|   IBIS model for TI tms320c6657_55 DSP
[IBIS Ver]   5.0
[Disclaimer]   Please be aware that in the absence of a written agreement
|   Texas Instruments(TI) assumes no liability for:
|   (1) The accuracy of the IBIS models provided to your company,
|   however, the IBIS model is compliant to industry standard
|   IQ Level 2a.  Refer to IBIS Quality Section below for
|   for full details.
|   (2) The proper functioning of these Models in your design
|   or for any resulting applications
|   (3) Infringement of patents, copyrights or intellectual
|   property rights resulting from your use of these
|   models.
|   TI provides IBIS Models as a service to our customers and
|   therefore reserves the right to limit distribution of the
|   Models.  The information is subject to change without notice.
[File Name]  tms320c6657_55_r1p2.ibs
[File Rev]   1.2
[Date]   18Sept2012
[Source]   Texas Instruments Incorporated
[Copyright]   Property of Texas Instruments Incorporated.
|   Unauthorized reproduction and/or distribution is strictly.
|   prohibited.
|   This product is protected under copyright law and trade
|   secret law as an unpublished work.
|   Created 2012,(C) Copyright 2010-2020,
|   Texas Instruments Incorporated., All Rights Reserved.
|   These commodities are under the U.S. Government
|   distribution license control. As such,they are not to be
|   re-exported without the prior approval of the U.S.
|   Department of Commerce.
[Notes]
   For SerDes simulations use Texas Instruments IBIS AMI models
   Some IV curves contain Non monotonic data points.
|   Model Generated by W.T.
|   Model Updated by R.L.
|   **For SerDes simulations use Texas Instruments IBIS AMI models**
| The DDR3
| Definitions:
| Drive strength defined by resistor value connected to PTV15 pin
|   9MA_FT9MA   : Full Termination Thevenin  [45 ohm] [45ohm to Vtt]
| Slew Rate Definitions:
| The Driver Slew Rate is defined by the value of the DDRSLRATE0 and
| DDRSLRATE1 pins.
|   FASTEST Slew Rate : SR1 0;SR0 0
|   FAST Slew Rate   : SR1 0;SR0 1
|   SLOW Slew Rate   : SR1 1;SR0 0
|   SLOWEST Slew Rate : SR1 1;SR0 1
| To choose the correct model, determine the settings of the DDRSLRATE[1:0]
| pins.  Look for the keyword from the tables above to select the proper
| models.  For example if the DDRSLRATE1 pin is pulled high and the
| DDRSLRATE0 pin is pulled low then the slew rate keyword is SLOW.  For
| this example the model needed for the address and control pins would be
| CSCDVG_SLOW_9MA, the data and DQM pins would be CSCDVG_SLOW_9MA_FT9MA and
| the DQS pins would be CSCDDVG_SLOW_9MA_FT9MA_N and CSCDDVG_SLOW_9MA_FT9MA_P.
|   Revision History
|   GERNERAL COMMENT: All IBIS Quality Notes below reflect latest release
|   and version of IBIS File
|   Revision 1.0 --14Feb 2012
|   -Initial Release
|   Revision 1.2 --18Sept 2012
|   -Updated pin list and naming conventions
|   File passes ibischk5.0 with 0 errors and 16 warnings
|   Model generated and correlated using HSPICE version 2005.09-SP1
|   IBIS Quality Notes
|IQ
|IQ Component tms320c6657: Overall Quality level 2a
|IQ
|IQ ibischk5 (5.0.7)
|IQ   -Parser for IBISCHK5 resulted in 16 warnings
|IQ   -8 warnings pertaining to typ/min/max values never becoming zero
|IQ   specific warnings identified by OP buffer type below
|IQ   -8 warnings pertaining to the Series Mosfet having decreasing current
|IQ   -Parser for IBISCHK5 resulted in muliple notes regarding non-monotonic data
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[Component] tms320c6657_55
[Manufacturer] Texas Instruments
[Package Model] 6657
[Package]
|Variable   Typ   Min   Max
R_pkg   1.0013   0.15483   2.0653
L_pkg   2.89689nH  0.94768nH   5.3815nH
C_pkg   1.63791pF  0.87102pF   2.5609pF
[Pin]  signal_name   model_name
A1   VSS   GND
A2   DDRDQS3P   DQS   |   bshtltcscddvgpbfz
A3   DDRD20   DQ   |   bshtltcscdvgpbfz
A4   DDRDQS2N   DQS   |   bshtltcscddvgpbfz
A5   DDRD11   DQ   |   bshtltcscdvgpbfz
A6   DDRD10   DQ   |   bshtltcscdvgpbfz
A7   DDRDQS1N   DQS   |   bshtltcscddvgpbfz
A8   DDRDQM0   DM   |   bshtltcscdvgpbfz
A9   DDRD00   DQ   |   bshtltcscdvgpbfz
A10   VSS   GND
A11   DDRD06   DQ   |   bshtltcscdvgpbfz
A12   DDRCB03   DQ   |   bshtltcscdvgpbfz
A13   DDRDQS8N   DQS   |   bshtltcscddvgpbfz
A14   DDRCLKOUTP0   CLK_OUT   |   bshtltcscdvgpbfz
A15   DDRRASZ   ACC_OUT   |   bshtltcscdvgpbfz
A16   DDRCKE0   ACC_OUT   |   bshtltcscdvgpbfz
A17   DDRA05   ACC_OUT   |   bshtltcscdvgpbfz
A18   DDRA07   ACC_OUT   |   bshtltcscdvgpbfz
A19   DDRA01   ACC_OUT   |   bshtltcscdvgpbfz
A20   DDRCKE1   ACC_OUT   |   bshtltcscdvgpbfz
A21   DDRCLKOUTP1   CLK_OUT   |   bshtltcscdvgpbfz
A22   DDRCLKP   iclkrx10g
A23   RSV07   NC
A24   DVDD18   POWER
A25   VSS   GND
B1   DDRD26   DQ   |   bshtltcscdvgpbfz
B2   DDRDQS3N   DQS   |   bshtltcscddvgpbfz
B3   DDRD17   DQ   |   bshtltcscdvgpbfz
B4   DDRDQS2P   DQS   |   bshtltcscddvgpbfz
B5   DDRD21   DQ   |   bshtltcscdvgpbfz
B6   VSS   GND
B7   DDRDQS1P   DQS   |   bshtltcscddvgpbfz
B8   DDRD15   DQ   |   bshtltcscdvgpbfz
B9   DDRD03   DQ   |   bshtltcscdvgpbfz
B10   DVDD15   POWER
B11   DDRD07   DQ   |   bshtltcscdvgpbfz
B12   DDRCB01   DQ   |   bshtltcscdvgpbfz
B13   DDRDQS8P   DQS   |   bshtltcscddvgpbfz
B14   DDRCLKOUTN0   CLK_OUT   |   bshtltcscdvgpbfz
B15   DDRCE0Z   ACC_OUT   |   bshtltcscdvgpbfz
B16   DDRRESETZ   ACC_OUT   |   bshtltcscdvgpbfz
B17   VSS   GND
B18   DDRA04   ACC_OUT   |   bshtltcscdvgpbfz
B19   DDRBA2   ACC_OUT   |   bshtltcscdvgpbfz
B20   DDRA11   ACC_OUT   |   bshtltcscdvgpbfz
B21   DDRCLKOUTN1   CLK_OUT   |   bshtltcscdvgpbfz
B22   DDRCLKN   iclkrx10g
B23   RSV06   NC
B24   MCMRXFLCLK   bc1850cghypbfb
B25   MCMCLKN   iclkrx10g
C1   DDRD27   DQ   |   bshtltcscdvgpbfz
C2   VSS   GND
C3   DDRD30   DQ   |   bshtltcscdvgpbfz
C4   VSS   GND
C5   DDRD22   DQ   |   bshtltcscdvgpbfz
C6   DVDD15   POWER
C7   DDRD13   DQ   |   bshtltcscdvgpbfz
C8   VSS   GND
C9   DDRD01   DQ   |   bshtltcscdvgpbfz
C10   DDRDQS0N   DQS   |   bshtltcscddvgpbfz
C11   DDRCB02   DQ   |   bshtltcscdvgpbfz
C12   DDRDQM8   DM   |   bshtltcscdvgpbfz
C13   VSS   GND
C14   DDRCE1Z   ACC_OUT   |   bshtltcscdvgpbfz
C15   VSS   GND
C16   DDRA06   ACC_OUT   |   bshtltcscdvgpbfz
C17   DVDD15   POWER
C18   DDRBA0   ACC_OUT   |   bshtltcscdvgpbfz
C19   VSS   GND
C20   DDRA13   ACC_OUT   |   bshtltcscdvgpbfz
C21   DVDD15   POWER
C22   DDRSLRATE0   bc1850cghypbfb
C23   RSV09   NC
C24   MCMRXFLDAT   bc1850cghypbfb
C25   MCMCLKP   iclkrx10g
D1   DDRD28   DQ   |   bshtltcscdvgpbfz
D2   DVDD15   POWER
D3   DDRD29   DQ   |   bshtltcscdvgpbfz
D4   DVDD15   POWER
D5   DDRD23   DQ   |   bshtltcscdvgpbfz
D6   DDRD12   DQ   |   bshtltcscdvgpbfz
D7   DDRD14   DQ   |   bshtltcscdvgpbfz
D8   DVDD15   POWER
D9   DDRD02   DQ   |   bshtltcscdvgpbfz
D10   DDRDQS0P   DQS   |   bshtltcscddvgpbfz
D11   DDRCB00   DQ   |   bshtltcscdvgpbfz
D12   DDRODT1   ACC_OUT   |   bshtltcscdvgpbfz
D13   DVDD15   POWER
D14   DDRCASZ   ACC_OUT   |   bshtltcscdvgpbfz
D15   DVDD15   POWER
D16   DDRA00   ACC_OUT   |   bshtltcscdvgpbfz
D17   DDRBA1   ACC_OUT   |   bshtltcscdvgpbfz
D18   DDRA12   ACC_OUT   |   bshtltcscdvgpbfz
D19   DVDD15   POWER
D20   DDRA08   ACC_OUT   |   bshtltcscdvgpbfz
D21   VSS   GND
D22   DDRSLRATE1   bc1850cghypbfb
D23   RSV21   NC
D24   MCMRXPMDAT   bc1850cghypbfb
D25   MCMTXFLDAT   bc1850cghypbfb
E1   DDRDQM3   DM   |   bshtltcscdvgpbfz
E2   DDRD24   DQ   |   bshtltcscdvgpbfz
E3   DDRD31   DQ   |   bshtltcscdvgpbfz
E4   DDRD19   DQ   |   bshtltcscdvgpbfz
E5   DDRD16   DQ   |   bshtltcscdvgpbfz
E6   DDRD08   DQ   |   bshtltcscdvgpbfz
E7   DDRDQM1   DM   |   bshtltcscdvgpbfz
E8   DDRD09   DQ   |   bshtltcscdvgpbfz
E9   DDRD04   DQ   |   bshtltcscdvgpbfz
E10   DDRD05   DQ   |   bshtltcscdvgpbfz
E11   VSS   GND
E12   VREFSSTL   NC
E13   DDRWEZ   ACC_OUT   |   bshtltcscdvgpbfz
E14   DDRODT0   ACC_OUT   |   bshtltcscdvgpbfz
E15   DDRA03   ACC_OUT   |   bshtltcscdvgpbfz
E16   DDRA02   ACC_OUT   |   bshtltcscdvgpbfz
E17   DDRA15   ACC_OUT   |   bshtltcscdvgpbfz
E18   DDRA14   ACC_OUT   |   bshtltcscdvgpbfz
E19   DDRA10   ACC_OUT   |   bshtltcscdvgpbfz
E20   DDRA09   ACC_OUT   |   bshtltcscdvgpbfz
E21   DVDD18   POWER
E22   VCNTL0   bi2c18gfz
E23   VCNTL1   bi2c18gfz
E24   MCMRXPMCLK   bc1850cghypbfb
E25   MCMTXFLCLK   bc1850cghypbfb
F1   LRESETNMIENZ   bc1850cghypbfb
F2   DDRD25   DQ   |   bshtltcscdvgpbfz
F3   VSS   GND
F4   DDRD18   DQ   |   bshtltcscdvgpbfz
F5   DDRDQM2   DM   |   bshtltcscdvgpbfz
F6   VSS   GND
F7   DVDD15   POWER
F8   VSS   GND
F9   DVDD15   POWER
F10   VSS   GND
F11   DVDD15   POWER
F12   VSS   GND
F13   DVDD15   POWER
F14   VSS   GND
F15   PTV15   NC
F16   VSS   GND
F17   DVDD15   POWER
F18   VSS   GND
F19   DVDD15   POWER
F20   AVDDA2   POWER
F21   RSV14   NC
F22   RSV20   NC
F23   VCNTL2   bi2c18gfz
F24   MCMTXPMCLK   bc1850cghypbfb
F25   MCMREFCLKOUTN   ocml10g
G1   EMIFCE1Z   bc1850cghypbfb
G2   HOUT   bc1840dghypbfb
G3   DVDD18   POWER
G4   LRESETZ   bc1850cghypbfb
G5   CORESEL1   bc1850cghypbfb
G6   DVDD18   POWER
G7   VSS   GND
G8   DVDD15   POWER
G9   VSS   GND
G10   DVDD15   POWER
G11   VSS   GND
G12   DVDD15   POWER
G13   VSS   GND
G14   DVDD15   POWER
G15   VSS   GND
G16   DVDD15   POWER
G17   VSS   GND
G18   DVDD15   POWER
G19   RSV0A   NC
G20   RSV0B   NC
G21   RSV15   NC
G22   RSV10   NC
G23   VCNTL3   bi2c18gfz
G24   MCMTXPMDAT   bc1850cghypbfb
G25   MCMREFCLKOUTP   ocml10g
H1   NMIZ   bc1850cghypbfb
H2   RSV03   NC
H3   BOOTCOMPLETE   bc1850cghypbfb
H4   RESETZ   ic18ghypbfb
H5   RESETSTATZ   bc1850cghypbfb
H6   VSS   GND
H7   DVDD18   POWER
H8   VSS   GND
H9   CVDD   POWER
H10   VSS   GND
H11   CVDD   POWER
H12   VSS   GND
H13   CVDD   POWER
H14   VSS   GND
H15   CVDD   POWER
H16   VSS   GND
H17   CVDD   POWER
H18   VSS   GND
H19   DVDD18   POWER
H20   VSS   GND
H21   VSS   GND
H22   RSV11   NC
H23   VSS   GND
H24   DVDD18   POWER
H25   VSS   GND
J1   EMIFBE0Z   bc1850cghypbfb
J2   EMIFCE2Z   bc1850cghypbfb
J3   RSV02   NC
J4   RESETFULLZ   ic18ghypbfb
J5   CORESEL0   bc1850cghypbfb
J6   DVDD18   POWER
J7   VSS   GND
J8   CVDD1   POWER
J9   VSS   GND
J10   CVDD   POWER
J11   VSS   GND
J12   CVDD   POWER
J13   VSS   GND
J14   CVDD   POWER
J15   VSS   GND
J16   CVDD   POWER
J17   VSS   GND
J18   CVDD1   POWER
J19   VSS   GND
J20   RSV16   NC
J21   MCMTXN3   NC
J22   VSS   GND
J23   VSS   GND
J24   VSS   GND
J25   MCMRXN2   NC
K1   EMIFA00   bc1850cghypbfb
K2   VSS   GND
K3   DVDD18   POWER
K4   EMIFWEZ   bc1850cghypbfb
K5   EMIFCE0Z   bc1850cghypbfb
K6   VSS   GND
K7   DVDD18   POWER
K8   VSS   GND
K9   CVDD1   POWER
K10   VSS   GND
K11   CVDD   POWER
K12   VSS   GND
K13   CVDD   POWER
K14   VSS   GND
K15   CVDD   POWER
K16   VSS   GND
K17   CVDD1   POWER
K18   VSS   GND
K19   VDDT1   POWER
K20   VSS   GND
K21   MCMTXP3   NC
K22   MCMTXN2   NC
K23   VSS   GND
K24   MCMRXN3   NC
K25   MCMRXP2   NC
L1   EMIFA04   bc1850cghypbfb
L2   EMIFA02   bc1850cghypbfb
L3   EMIFBE1Z   bc1850cghypbfb
L4   EMIFOEZ   bc1850cghypbfb
L5   EMIFRNW   bc1850cghypbfb
L6   DVDD18   POWER
L7   VSS   GND
L8   CVDD   POWER
L9   VSS   GND
L10   CVDD   POWER
L11   VSS   GND
L12   CVDD   POWER
L13   VSS   GND
L14   CVDD   POWER
L15   VSS   GND
L16   CVDD   POWER
L17   VSS   GND
L18   CVDD   POWER
L19   VSS   GND
L20   VDDT1   POWER
L21   VSS   GND
L22   MCMTXP2   NC
L23   VSS   GND
L24   MCMRXP3   NC
L25   VSS   GND
M1   EMIFA07   bc1850cghypbfb
M2   EMIFA06   bc1850cghypbfb
M3   EMIFA01   bc1850cghypbfb
M4   EMIFWAIT1   bc1850cghypbfb
M5   EMIFCE3Z   bc1850cghypbfb
M6   VSS   GND
M7   DVDD18   POWER
M8   VSS   GND
M9   CVDD   POWER
M10   VSS   GND
M11   CVDD   POWER
M12   VSS   GND
M13   CVDD   POWER
M14   VSS   GND
M15   CVDD   POWER
M16   VSS   GND
M17   CVDD   POWER
M18   VSS   GND
M19   VDDT1   POWER
M20   VDDR1   POWER
M21   MCMTXP1   NC
M22   VSS   GND
M23   VSS   GND
M24   VSS   GND
M25   MCMRXN1   NC
N1   EMIFA10   bc1850cghypbfb
N2   EMIFA08   bc1850cghypbfb
N3   DVDD18   POWER
N4   VSS   GND
N5   EMIFWAIT0   bc1850cghypbfb
N6   DVDD18   POWER
N7   VSS   GND
N8   CVDD   POWER
N9   VSS   GND
N10   CVDD   POWER
N11   VSS   GND
N12   CVDD   POWER
N13   VSS   GND
N14   CVDD   POWER
N15   VSS   GND
N16   CVDD   POWER
N17   VSS   GND
N18   CVDD   POWER
N19   VSS   GND
N20   VDDT1   POWER
N21   MCMTXN1   NC
N22   MCMTXP0   NC
N23   VSS   GND
N24   MCMRXP0   NC
N25   MCMRXP1   NC
P1   EMIFA12   bc1850cghypbfb
P2   EMIFA11   bc1850cghypbfb
P3   EMIFA09   bc1850cghypbfb
P4   EMIFA05   bc1850cghypbfb
P5   EMIFA03   bc1850cghypbfb
P6   VSS   GND
P7   DVDD18   POWER
P8   VSS   GND
P9   CVDD   POWER
P10   VSS   GND
P11   CVDD   POWER
P12   VSS   GND
P13   CVDD   POWER
P14   VSS   GND
P15   CVDD   POWER
P16   VSS   GND
P17   CVDD   POWER
P18   VSS   GND
P19   CVDD   POWER
P20   VSS   GND
P21   VSS   GND
P22   MCMTXN0   NC
P23   VSS   GND
P24   MCMRXN0   NC
P25   VSS   GND
R1   EMIFA17   bc1850cghypbfb
R2   EMIFA16   bc1850cghypbfb
R3   EMIFA14   bc1850cghypbfb
R4   EMIFA15   bc1850cghypbfb
R5   EMIFA13   bc1850cghypbfb
R6   DVDD18   POWER
R7   VSS   GND
R8   VSS   GND
R9   VSS   GND
R10   CVDD   POWER
R11   VSS   GND
R12   CVDD   POWER
R13   VSS   GND
R14   CVDD   POWER
R15   VSS   GND
R16   CVDD   POWER
R17   VSS   GND
R18   CVDD   POWER
R19   VSS   GND
R20   DVDD18   POWER
R21   GPIO07   bc1840dghypbfb
R22   VSS   GND
R23   GPIO02   bc1840dghypbfb
R24   VSS   GND
R25   GPIO01   bc1840dghypbfb
T1   EMIFA19   bc1850cghypbfb
T2   VSS   GND
T3   DVDD18   POWER
T4   EMIFA18   bc1850cghypbfb
T5   EMIFA20   bc1850cghypbfb
T6   VSS   GND
T7   DVDD18   POWER
T8   VSS   GND
T9   CVDD1   POWER
T10   VSS   GND
T11   CVDD   POWER
T12   VSS   GND
T13   CVDD   POWER
T14   VSS   GND
T15   CVDD   POWER
T16   VSS   GND
T17   CVDD1   POWER
T18   VSS   GND
T19   DVDD18   POWER
T20   VSS   GND
T21   GPIO12   bc1840dghypbfb
T22   GPIO06   bc1840dghypbfb
T23   GPIO04   bc1840dghypbfb
T24   DVDD18   POWER
T25   GPIO00   bc1840dghypbfb
U1   EMIFA21   bc1850cghypbfb
U2   EMIFA22   bc1850cghypbfb
U3   EMIFA23   bc1850cghypbfb
U4   EMIFD00   bc1850cghypbfb
U5   EMIFD01   bc1850cghypbfb
U6   DVDD18   POWER
U7   VSS   GND
U8   CVDD1   POWER
U9   VSS   GND
U10   CVDD   POWER
U11   VSS   GND
U12   CVDD   POWER
U13   VSS   GND
U14   CVDD   POWER
U15   VSS   GND
U16   CVDD   POWER
U17   VSS   GND
U18   CVDD1   POWER
U19   VSS   GND
U20   DVDD18   POWER
U21   GPIO11   bc1840dghypbfb
U22   GPIO08   bc1840dghypbfb
U23   GPIO09   bc1840dghypbfb
U24   GPIO05   bc1840dghypbfb
U25   GPIO03   bc1840dghypbfb
V1   EMIFD02   bc1850cghypbfb
V2   EMIFD03   bc1850cghypbfb
V3   EMIFD04   bc1850cghypbfb
V4   EMIFD05   bc1850cghypbfb
V5   EMIFD07   bc1850cghypbfb
V6   VSS   GND
V7   DVDD18   POWER
V8   VSS   GND
V9   CVDD   POWER
V10   VSS   GND
V11   CVDD   POWER
V12   VSS   GND
V13   CVDD   POWER
V14   VSS   GND
V15   CVDD   POWER
V16   VSS   GND
V17   CVDD   POWER
V18   VSS   GND
V19   DVDD18   POWER
V20   VSS   GND
V21   GPIO15   bc1840dghypbfb
V22   GPIO13   bc1840dghypbfb
V23   GPIO10   bc1840dghypbfb
V24   EMU00   bc1840dghypbfb
V25   EMU01   bc1840dghypbfb
W1   EMIFD06   bc1850cghypbfb
W2   EMIFD08   bc1850cghypbfb
W3   VSS   GND
W4   EMIFD10   bc1850cghypbfb
W5   EMIFD12   bc1850cghypbfb
W6   DVDD18   POWER
W7   VSS   GND
W8   VDDT2   POWER
W9   VSS   GND
W10   VDDT2   POWER
W11   VSS   GND
W12   VDDT2   POWER
W13   VSS   GND
W14   DVDD18   POWER
W15   VSS   GND
W16   DVDD18   POWER
W17   VSS   GND
W18   DVDD18   POWER
W19   VSS   GND
W20   DVDD18   POWER
W21   GPIO14   bc1840dghypbfb
W22   EMU08   bc1840dghypbfb
W23   EMU03   bc1840dghypbfb
W24   EMU04   bc1840dghypbfb
W25   EMU02   bc1840dghypbfb
Y1   EMIFD09   bc1850cghypbfb
Y2   EMIFD11   bc1850cghypbfb
Y3   DVDD18   POWER
Y4   RSV13   NC
Y5   RSV12   NC
Y6   VSS   GND
Y7   VDDT2   POWER
Y8   VSS   GND
Y9   VDDT2   POWER
Y10   VSS   GND
Y11   VDDT2   POWER
Y12   VSS   GND
Y13   DVDD18   POWER
Y14   VSS   GND
Y15   AVDDA1   POWER
Y16   VSS   GND
Y17   DVDD18   POWER
Y18   PORZ   ihhv18g
Y19   RSV08   NC
Y20   CLKX0   bc1850cghypbfb
Y21   EMU18   bc1840dghypbfb
Y22   EMU09   bc1840dghypbfb
Y23   EMU07   bc1840dghypbfb
Y24   EMU06   bc1840dghypbfb
Y25   EMU05   bc1840dghypbfb
AA1   EMIFD13   bc1850cghypbfb
AA2   EMIFD15   bc1850cghypbfb
AA3   VDDR3   POWER
AA4   VSS   GND
AA5   VDDR4   POWER
AA6   VSS   GND
AA7   RSV17   NC
AA8   VSS   GND
AA9   VDDR2   POWER
AA10   VSS   GND
AA11   RSV18   NC
AA12   SPISCS0   bc1850cghypbfb
AA13   SPICLK   bc1850cghypbfb
AA14   SPISCS1   bc1850cghypbfb
AA15   UARTTXD   bc1850cghypbfb
AA16   MDCLK   bc1850cghypbfb
AA17   SCL   bi2c18gfz
AA18   SDA   bi2c18gfz
AA19   SYSCLKOUT   bc1850cghypbfb
AA20   FSX0   bc1850cghypbfb
AA21   CLKR0   bc1850cghypbfb
AA22   RSV01   NC
AA23   EMU14   bc1840dghypbfb
AA24   EMU10   bc1840dghypbfb
AA25   EMU11   bc1840dghypbfb
AB1   EMIFD14   bc1850cghypbfb
AB2   VSS   GND
AB3   RSV19   NC
AB4   RIOTXN3   NC
AB5   RIOTXP3   NC
AB6   VSS   GND
AB7   RIOTXN1   NC
AB8   RIOTXP1   NC
AB9   VSS   GND
AB10   PCIETXP1   NC
AB11   PCIETXN1   NC
AB12   VSS   GND
AB13   SPIDOUT   bc1850cghypbfb
AB14   SPIDIN   bc1850cghypbfb
AB15   UARTRXD   bc1850cghypbfb
AB16   MDIO   bc1850cghypbfb
AB17   UARTRTS   bc1850cghypbfb
AB18   RSV05   NC
AB19   TRSTZ   ic18ghypbfb
AB20   VSS   GND
AB21   DR0   bc1850cghypbfb
AB22   EMU15   bc1840dghypbfb
AB23   DVDD18   POWER
AB24   VSS   GND
AB25   EMU12   bc1840dghypbfb
AC1   VSS   GND
AC2   SGMII0TXN   NC
AC3   SGMII0TXP   NC
AC4   VSS   GND
AC5   RIOTXN2   NC
AC6   RIOTXP2   NC
AC7   VSS   GND
AC8   RIOTXP0   NC
AC9   RIOTXN0   NC
AC10   VSS   GND
AC11   PCIETXP0   NC
AC12   PCIETXN0   NC
AC13   VSS   GND
AC14   UARTRXD1   bc1850cghypbfb
AC15   UARTTXD1   bc1850cghypbfb
AC16   DVDD18   POWER
AC17   UARTCTS   bc1850cghypbfb
AC18   RSV04   NC
AC19   TIMO0   bc1850cghypbfb
AC20   DVDD18   POWER
AC21   CLKS1   bc1850cghypbfb
AC22   DX0   bc1850cghypbfb
AC23   CLKS0   bc1850cghypbfb
AC24   EMU17   bc1840dghypbfb
AC25   EMU13   bc1840dghypbfb
AD1   VSS   GND
AD2   VSS   GND
AD3   VSS   GND
AD4   RIORXN3   NC
AD5   RIORXP3   NC
AD6   VSS   GND
AD7   RIORXP1   NC
AD8   RIORXN1   NC
AD9   VSS   GND
AD10   PCIERXN1   NC
AD11   PCIERXP1   NC
AD12   VSS   GND
AD13   SRIOSGMIICLKP   iclkrx10g
AD14   PCIECLKP   iclkrx10g
AD15   UARTRTS1   bc1850cghypbfb
AD16   VSS   GND
AD17   TCK   ic18ghypbfb
AD18   CORECLKP   iclkrx10g
AD19   TDO   bc1840dghypbfb
AD20   TIMI0   bc1850cghypbfb
AD21   DR1   bc1850cghypbfb
AD22   FSR1   bc1850cghypbfb
AD23   CLKR1   bc1850cghypbfb
AD24   FSR0   bc1850cghypbfb
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|********************  DIFF PIN  *******************************
[Diff_pin]  inv_pin   vdiff  tdelay_typ  tdelay_min  tdelay_max
A14   B14   200mV   NA   NA   NA   || DDRCLKOUTP0 & DDRCLKOUTN0
A21   B21   200mV   NA   NA   NA   || DDRCLKOUTP1 & DDRCLKOUTN1
D10   C10   200mV   NA   NA   NA   || DDRDQS0P & DDRDQS0N
B7   A7   200mV   NA   NA   NA   || DDRDQS1P & DDRDQS1N
B4   A4   200mV   NA   NA   NA   || DDRDQS2P & DDRDQS2N
A2   B2   200mV   NA   NA   NA   || DDRDQS3P & DDRDQS3N
B13   A13   200mV   NA   NA   NA   || DDRDQS8P & DDRDQS8N
AD18   AE19   NA   NA   NA   NA   || CORECLKP & CORECLKN
A22   B22   NA   NA   NA   NA   || DDRCLKP & DDRCLKN
C25   B25   NA   NA   NA   NA   || MCMCLKP & MCMCLKN
AD14   AE15   NA   NA   NA   NA   || PCIECLKP & PCIECLKN
AD13   AE14   NA   NA   NA   NA   || SRIOSGMIICLKP & SRIOSGMIICLKN
G25   F25   50mV   NA   NA   NA   || MCMREFCLKOUTP & MCMREFCLKOUTN
[Model Selector] ocml10g
|ocml10g   [30Jul2010 Revision 1.0]
ocml10g_0p9 Model operating at 0.9V nom VDDS
|ocml10g_0p9;
ocml10g_1   Model operating at 1V nom VDDS
|ocml10g_1;
[Model Selector] bc1840dghypbfb
|bc1840dghypbfb.ibs   [15July11 revision 1.0]
BC1840DGHYPBFB_WK_PD  Cell operated at 1.8(nom)
|IO in Rx mode with weak pulldown on in 1.8V mode
BC1840DGHYPBFB_WK_PU  Cell operated at 1.8(nom)
|IO in Rx mode with weak pullup on  in 1.8V mode
BC1840DGHYPBFB_DRIVER_MODE  Cell operated at 1.8(nom)
|Normal IO mode of operation at 1.8V VDDS
[Model Selector] bc1850cghypbfb
|bc1850cghypbfb.ibs [15July2011 revision 1.0]
BC1850CGHYPBFB_WK_PD  Cell operated at 1.8(nom)
|IO in Rx mode with weak pulldown on  in 1.8V mode
BC1850CGHYPBFB_WK_PU  Cell operated at 1.8(nom)
|IO in Rx mode with weak pullup on in 1.8V mode
BC1850CGHYPBFB_DRIVER_MODE  Cell operated at 1.8(nom)
|   DDR ACC
[Model Selector]   ACC_OUT
| bshtltcscdvg.ibs   [6 Sep 2011 Revision 1.6]
CSCDVG_SLOWEST_9MA   TX 45 ohms Slowest (SR1 1; SR0 1)
CSCDVG_SLOW_9MA   TX 45 ohms Slow (SR1 1; SR0 0)
CSCDVG_FAST_9MA   TX 45 ohms Fast (SR1 0; SR0 1)
CSCDVG_FASTEST_9MA   TX 45 ohms Fastest (SR1 0; SR0 0)
|   DDR CLOCK_OUT
[Model Selector]   CLK_OUT
| bshtltcscdvg.ibs   [6 Sep 2011 Revision 1.6]
CSCDVG_SLOWEST_9MA   TX 45 ohms Slowest (SR1 1; SR0 1)
CSCDVG_SLOW_9MA   TX 45 ohms Slow (SR1 1; SR0 0)
CSCDVG_FAST_9MA   TX 45 ohms Fast (SR1 0; SR0 1)
CSCDVG_FASTEST_9MA   TX 45 ohms Fastest (SR1 0; SR0 0)
|   DDR DQ
[Model Selector] DQ
| bshtltcscdvg.ibs   [6 Sep 2011 Revision 1.6]
CSCDVG_SLOWEST_9MA_FT9MA   Cell operated at 1.5(nom)
CSCDVG_SLOW_9MA_FT9MA   Cell operated at 1.5(nom)
CSCDVG_FAST_9MA_FT9MA   Cell operated at 1.5(nom)
CSCDVG_FASTEST_9MA_FT9MA   Cell operated at 1.5(nom)
|   DDR DQM
[Model Selector] DM
| bshtltcscdvg.ibs   [6 Sep 2011 Revision 1.6]
CSCDVG_SLOWEST_9MA_FT9MA   Cell operated at 1.5(nom)
CSCDVG_SLOW_9MA_FT9MA   Cell operated at 1.5(nom)
CSCDVG_FAST_9MA_FT9MA   Cell operated at 1.5(nom)
CSCDVG_FASTEST_9MA_FT9MA   Cell operated at 1.5(nom)
|   DDR DQS
| Negative Pad
[Model Selector] DQS
| bshtltcscddvg.ibs   [6 Sep 2011 Revision 1.6]
CSCDDVG_SLOWEST_9MA_FT9MA_N   Cell operated at 1.5(nom)
CSCDDVG_SLOW_9MA_FT9MA_N   Cell operated at 1.5(nom)
CSCDDVG_FAST_9MA_FT9MA_N   Cell operated at 1.5(nom)
CSCDDVG_FASTEST_9MA_FT9MA_N   Cell operated at 1.5(nom)
|   DDR DQS
| Positive Pad
CSCDDVG_SLOWEST_9MA_FT9MA_P   Cell operated at 1.5(nom)
CSCDDVG_SLOW_9MA_FT9MA_P   Cell operated at 1.5(nom)
CSCDDVG_FAST_9MA_FT9MA_P   Cell operated at 1.5(nom)
CSCDDVG_FASTEST_9MA_FT9MA_P   Cell operated at 1.5(nom)
[Model Selector] ic18ghypbfb
| ic18ghypbfb.ibs  [11July2011 revision 1.0]
IC18GHYPBFB_WK_PD_ON   Cell operated at 1.8(nom)
IC18GHYPBFB_WK_PU_ON   Cell operated at 1.8(nom)
IC18GHYPBFB_RX_MODE   Cell operated at 1.8(nom)
[Model Selector] iclkrx10g
iclkrx10g_0p9 Cell operated at 0p9(nom)
| iclkrx10g_0p9.ibs  [08Jul11 revision 1.3]
s_iclkrx10g_0p9 Cell operated at 0p9(nom)
| iclkrx10g_0p9.ibs  [08Jul11 revision 1.3]
iclkrx10g_1 Cell operated at 1p0(nom)
| iclkrx10g_1.ibs  [08Jul11 revision 1.2]
s_iclkrx10g_1 Cell operated at 1p0(nom)
|   Package Model Definition
[Define Package Model]  6657
[Manufacturer]   Texas Instruments Incorporated
[OEM]   Texas Instruments Incorporated
[Description]   Package for tms320c6657_55
[Number Of Pins]   323
[Pin Numbers]
H3   | 1 BGA-H3 BOOTCOMPLETE
G2   | 2 BGA-G2 HOUT
J4   | 3 BGA-J4 RESETFULLZ
AA21 | 4 BGA-AA21 CLKR0
AC23 | 5 BGA-AC23 CLKS0
Y20  | 6 BGA-Y20 CLKX0
AD23 | 7 BGA-AD23 CLKR1
AE24 | 8 BGA-AE24 CLKX1
AC22 | 9 BGA-AC22 DX0
AD24 | 10 BGA-AD24 FSR0
AC21 | 11 BGA-AC21 CLKS1
AD22 | 12 BGA-AD22 FSR1
Y21  | 13 BGA-Y21 EMU18
AE15 | 14 BGA-AE15 PCIECLKN
AD14 | 15 BGA-AD14 PCIECLKP
AC14 | 16 BGA-AC14 UARTRXD1
Y19  | 17 BGA-Y19 RSV08
AA19 | 18 BGA-AA19 SYSCLKOUT
Y18  | 19 BGA-Y18 PORZ
AB18 | 20 BGA-AB18 RSV05
AC18 | 21 BGA-AC18 RSV04
AB19 | 22 BGA-AB19 TRSTZ
J5   | 23 BGA-J5 CORESEL0
H5   | 24 BGA-H5 RESETSTATZ
G5   | 25 BGA-G5 CORESEL1
G4   | 26 BGA-G4 LRESETZ
C23  | 27 BGA-C23 RSV09
C22  | 28 BGA-C22 DDRSLRATE0
B22  | 29 BGA-B22 DDR3CLKN
A22  | 30 BGA-A22 DDR3CLKP
A23  | 31 BGA-A23 RSV07
D16  | 32 BGA-D16 DDRA00
B18  | 33 BGA-B18 DDRA04
E15  | 34 BGA-E15 DDRA03
A19  | 35 BGA-A19 DDRA01
E16  | 36 BGA-E16 DDRA02
D17  | 37 BGA-D17 DDRBA1
A18  | 38 BGA-A18 DDRA07
A17  | 39 BGA-A17 DDRA05
C16  | 40 BGA-C16 DDRA06
B16  | 41 BGA-B16 DDRRESETZ
D20  | 42 BGA-D20 DDRA08
E20  | 43 BGA-E20 DDRA09
E19  | 44 BGA-E19 DDRA10
B20  | 45 BGA-B20 DDRA11
C20  | 46 BGA-C20 DDRA13
A21  | 47 BGA-A21 DDRCLKOUTP1
D18  | 48 BGA-D18 DDRA12
E18  | 49 BGA-E18 DDRA14
E17  | 50 BGA-E17 DDRA15
A20  | 51 BGA-A20 DDRCKE1
C18  | 52 BGA-C18 DDRBA0
B19  | 53 BGA-B19 DDRBA2
D14  | 54 BGA-D14 DDRCASZ
C14  | 55 BGA-C14 DDRCE1Z
A15  | 56 BGA-A15 DDRRASZ
D11  | 57 BGA-D11 DDRCB00
C12  | 58 BGA-C12 DDRDQM8
C11  | 59 BGA-C11 DDRCB02
B12  | 60 BGA-B12 DDRCB01
A12  | 61 BGA-A12 DDRCB03
A13  | 62 BGA-A13 DDRDQS8N
B15  | 63 BGA-B15 DDRCE0Z
A16  | 64 BGA-A16 DDRCKE0
B23  | 65 BGA-B23 RSV06
B14  | 66 BGA-B14 DDRCLKOUTN0
A14  | 67 BGA-A14 DDRCLKOUTP0
B21  | 68 BGA-B21 DDRCLKOUTN1
A9   | 69 BGA-A9 DDRD00
A8   | 70 BGA-A8 DDRDQM0
B9   | 71 BGA-B9 DDRD03
C9   | 72 BGA-C9 DDRD01
D9   | 73 BGA-D9 DDRD02
D10  | 74 BGA-D10 DDRDQS0P
E9   | 75 BGA-E9 DDRD04
E10  | 76 BGA-E10 DDRD05
C10  | 77 BGA-C10 DDRDQS0N
A11  | 78 BGA-A11 DDRD06
B11  | 79 BGA-B11 DDRD07
E6   | 80 BGA-E6 DDRD08
E7   | 81 BGA-E7 DDRDQM1
D6   | 82 BGA-D6 DDRD12
E8   | 83 BGA-E8 DDRD09
A6   | 84 BGA-A6 DDRD10
A5   | 85 BGA-A5 DDRD11
A7   | 86 BGA-A7 DDRDQS1N
C7   | 87 BGA-C7 DDRD13
D7   | 88 BGA-D7 DDRD14
B8   | 89 BGA-B8 DDRD15
B7   | 90 BGA-B7 DDRDQS1P
E5   | 91 BGA-E5 DDRD16
F4   | 92 BGA-F4 DDRD18
F5   | 93 BGA-F5 DDRDQM2
B3   | 94 BGA-B3 DDRD17
A3   | 95 BGA-A3 DDRD20
E4   | 96 BGA-E4 DDRD19
B4   | 97 BGA-B4 DDRDQS2P
B5   | 98 BGA-B5 DDRD21
C5   | 99 BGA-C5 DDRD22
D5   | 100 BGA-D5 DDRD23
E2   | 101 BGA-E2 DDRD24
D1   | 102 BGA-D1 DDRD28
E1   | 103 BGA-E1 DDRDQM3
F2   | 104 BGA-F2 DDRD25
B1   | 105 BGA-B1 DDRD26
C1   | 106 BGA-C1 DDRD27
B2   | 107 BGA-B2 DDRDQS3N
D3   | 108 BGA-D3 DDRD29
E3   | 109 BGA-E3 DDRD31
C3   | 110 BGA-C3 DDRD30
A4   | 111 BGA-A4 DDRDQS2N
A2   | 112 BGA-A2 DDRDQS3P
B13  | 113 BGA-B13 DDRDQS8P
E14  | 114 BGA-E14 DDRODT0
E13  | 115 BGA-E13 DDRWEZ
D12  | 116 BGA-D12 DDRODT1
D22  | 117 BGA-D22 DDRSLRATE1
J3   | 118 BGA-J3 RSV02
H2   | 119 BGA-H2 RSV03
L5   | 120 BGA-L5 EMIFRNW
AB21 | 121 BGA-AB21 DR0
AA20 | 122 BGA-AA20 FSX0
AD21 | 123 BGA-AD21 DR1
AE22 | 124 BGA-AE22 DX1
AE23 | 125 BGA-AE23 FSX1
AE21 | 126 BGA-AE21 TIMI1
K1   | 127 BGA-K1 EMIFA00
L2   | 128 BGA-L2 EMIFA02
N5   | 129 BGA-N5 EMIFWAIT0
M3   | 130 BGA-M3 EMIFA01
P5   | 131 BGA-P5 EMIFA03
L1   | 132 BGA-L1 EMIFA04
M2   | 133 BGA-M2 EMIFA06
P4   | 134 BGA-P4 EMIFA05
M1   | 135 BGA-M1 EMIFA07
N2   | 136 BGA-N2 EMIFA08
P3   | 137 BGA-P3 EMIFA09
N1   | 138 BGA-N1 EMIFA10
P2   | 139 BGA-P2 EMIFA11
P1   | 140 BGA-P1 EMIFA12
R5   | 141 BGA-R5 EMIFA13
R4   | 142 BGA-R4 EMIFA15
R3   | 143 BGA-R3 EMIFA14
R2   | 144 BGA-R2 EMIFA16
R1   | 145 BGA-R1 EMIFA17
T1   | 146 BGA-T1 EMIFA19
T4   | 147 BGA-T4 EMIFA18
T5   | 148 BGA-T5 EMIFA20
U1   | 149 BGA-U1 EMIFA21
U2   | 150 BGA-U2 EMIFA22
U3   | 151 BGA-U3 EMIFA23
U4   | 152 BGA-U4 EMIFD00
J1   | 153 BGA-J1 EMIFBE0Z
L3   | 154 BGA-L3 EMIFBE1Z
M4   | 155 BGA-M4 EMIFWAIT1
K5   | 156 BGA-K5 EMIFCE0Z
K4   | 157 BGA-K4 EMIFWEZ
G1   | 158 BGA-G1 EMIFCE1Z
J2   | 159 BGA-J2 EMIFCE2Z
L4   | 160 BGA-L4 EMIFOEZ
M5   | 161 BGA-M5 EMIFCE3Z
U5   | 162 BGA-U5 EMIFD01
V1   | 163 BGA-V1 EMIFD02
V2   | 164 BGA-V2 EMIFD03
V3   | 165 BGA-V3 EMIFD04
V4   | 166 BGA-V4 EMIFD05
V5   | 167 BGA-V5 EMIFD07
W1   | 168 BGA-W1 EMIFD06
W2   | 169 BGA-W2 EMIFD08
Y1   | 170 BGA-Y1 EMIFD09
Y2   | 171 BGA-Y2 EMIFD11
W4   | 172 BGA-W4 EMIFD10
W5   | 173 BGA-W5 EMIFD12
AA1  | 174 BGA-AA1 EMIFD13
AB1  | 175 BGA-AB1 EMIFD14
AA2  | 176 BGA-AA2 EMIFD15
Y5   | 177 BGA-Y5 RSV12
V24  | 178 BGA-V24 EMU00
V25  | 179 BGA-V25 EMU01
V21  | 180 BGA-V21 GPIO15
W25  | 181 BGA-W25 EMU02
W24  | 182 BGA-W24 EMU04
W23  | 183 BGA-W23 EMU03
Y25  | 184 BGA-Y25 EMU05
Y24  | 185 BGA-Y24 EMU06
Y23  | 186 BGA-Y23 EMU07
W22  | 187 BGA-W22 EMU08
Y22  | 188 BGA-Y22 EMU09
AA24 | 189 BGA-AA24 EMU10
AA25 | 190 BGA-AA25 EMU11
AB25 | 191 BGA-AB25 EMU12
AC25 | 192 BGA-AC25 EMU13
AA23 | 193 BGA-AA23 EMU14
AD25 | 194 BGA-AD25 EMU16
AB22 | 195 BGA-AB22 EMU15
AA22 | 196 BGA-AA22 EMU19
AC24 | 197 BGA-AC24 EMU17
T25  | 198 BGA-T25 GPIO00
R25  | 199 BGA-R25 GPIO01
R23  | 200 BGA-R23 GPIO02
N25 | 201 BGA-N25 MCMRXN0
U25  | 202 BGA-U25 GPIO03
U24  | 203 BGA-U24 GPIO05
T23  | 204 BGA-T23 GPIO04
R21  | 205 BGA-R21 GPIO07
T22  | 206 BGA-T22 GPIO06
U23  | 207 BGA-U23 GPIO09
U22  | 208 BGA-U22 GPIO08
V23  | 209 BGA-V23 GPIO10
U21  | 210 BGA-U21 GPIO11
T21  | 211 BGA-T21 GPIO12
V22  | 212 BGA-V22 GPIO13
W21  | 213 BGA-W21 GPIO14
F1   | 214 BGA-F1 LRESETNMIENZ
H1   | 215 BGA-H1 NMIZ
H4   | 216 BGA-H4 RESETZ
J20 | 217 BGA-J20 MCMAMUX
K22 | 218 BGA-K22 MCMTXN3
J21 | 219 BGA-J21 MCMTXN2
B25 | 220 BGA-B25 MCMCLKN
C25 | 221 BGA-C25 MCMCLKP
B24 | 222 BGA-B24 MCMRXFLCLK
F25 | 223 BGA-F25 MCMREFCLKOUTN
G25 | 224 BGA-G25 MCMREFCLKOUTP
C24 | 225 BGA-C24 MCMRXFLDAT
E24 | 226 BGA-E24 MCMRXPMCLK
M25 | 227 BGA-M25 MCMRXP0
N24 | 228 BGA-N24 MCMRXN1
P24 | 229 BGA-P24 MCMRXP1
N21 | 230 BGA-N21 MCMTXN1
K24 | 231 BGA-K24 MCMRXN2
L24 | 232 BGA-L24 MCMRXP2
J25 | 233 BGA-J25 MCMRXN3
K25 | 234 BGA-K25 MCMRXP3
P22 | 235 BGA-P22 MCMTXN0
N22 | 236 BGA-N22 MCMTXP0
M21 | 237 BGA-M21 MCMTXP1
D24 | 238 BGA-D24 MCMRXPMDAT
F24 | 239 BGA-F24 MCMTXPMCLK
E25 | 240 BGA-E25 MCMTXFLCLK
D25 | 241 BGA-D25 MCMTXFLDAT
G24 | 242 BGA-G24 MCMTXPMDAT
K21 | 243 BGA-K21 MCMTXP2
L22 | 244 BGA-L22 MCMTXP3
AA16 | 245 BGA-AA16 MDCLK
AB16 | 246 BGA-AB16 MDIO
AA3  | 247 BGA-AA3 VDDR3
AA11 | 248 BGA-AA11 RSV18
AC12 | 249 BGA-AC12 PCIETXN0
AA12 | 250 BGA-AA12 SPISCS0
AD15 | 251 BGA-AD15 UARTRTS1
AE12 | 252 BGA-AE12 PCIERXN0
AE11 | 253 BGA-AE11 PCIERXP0
AC11 | 254 BGA-AC11 PCIETXP0
AD10 | 255 BGA-AD10 PCIERXN1
AD11 | 256 BGA-AD11 PCIERXP1
AB11 | 257 BGA-AB11 PCIETXN1
AB10 | 258 BGA-AB10 PCIETXP1
AC9 | 259 BGA-AC9 RIOTXN0
G22  | 260 BGA-G22 RSV10
H22  | 261 BGA-H22 RSV11
G21  | 262 BGA-G21 RSV15
AC19 | 263 BGA-AC19 TIMO0
F15  | 264 BGA-F15 PTV15
E12  | 265 BGA-E12 VREFSSTL
AE9 | 266 BGA-AE9 RIORXN0
AE8 | 267 BGA-AE8 RIORXP0
AD7 | 268 BGA-AD7 RIORXP1
AD8 | 269 BGA-AD8 RIORXN1
AE5 | 270 BGA-AE5 RIORXN2
AE6 | 271 BGA-AE6 RIORXP2
AD5 | 272 BGA-AD5 RIORXP3
AD4 | 273 BGA-AD4 RIORXN3
AC6 | 274 BGA-AC6 RIOTXP2
AC8 | 275 BGA-AC8 RIOTXP0
AB7 | 276 BGA-AB7 RIOTXN1
AB8 | 277 BGA-AB8 RIOTXP1
AC5 | 278 BGA-AC5 RIOTXN2
AB5 | 279 BGA-AB5 RIOTXP3
AB4 | 280 BGA-AB4 RIOTXN3
AA5  | 281 BGA-AA5 VDDR4
AA17 | 282 BGA-AA17 SCL
AA18 | 283 BGA-AA18 SDA
AB17 | 284 BGA-AB17 UARTRTS
AE18 | 285 BGA-AE18 TMS
AB3  | 286 BGA-AB3 RSV19
AA7  | 287 BGA-AA7 RSV17
AC2 | 288 BGA-AC2 SGMIITXN0
AE2 | 289 BGA-AE2 SGMIIRXN0
AE3 | 290 BGA-AE3 SGMIIRXP0
AC3 | 291 BGA-AC3 SGMIITXP0
AA13 | 292 BGA-AA13 SPICLK
AA14 | 293 BGA-AA14 SPISCS1
AC15 | 294 BGA-AC15 UARTTXD1
AB13 | 295 BGA-AB13 SPISIMO
AB14 | 296 BGA-AB14 SPISOMI
AE14 | 297 BGA-AE14 SRIOSGMIICLKN
AD13 | 298 BGA-AD13 SRIOSGMIICLKP
AE19 | 299 BGA-AE19 CORECLKN
AD18 | 300 BGA-AD18 CORECLKP
AD19 | 301 BGA-AD19 TDO
Y4   | 302 BGA-Y4 RSV13
F21  | 303 BGA-F21 RSV14
AD20 | 304 BGA-AD20 TIMI0
AE20 | 305 BGA-AE20 TIMO1
AC17 | 306 BGA-AC17 UARTCTS
AA15 | 307 BGA-AA15 UARTTXD
AE17 | 308 BGA-AE17 TDI
AD17 | 309 BGA-AD17 TCK
AB15 | 310 BGA-AB15 UARTRXD
AE16 | 311 BGA-AE16 UARTCTS1
M20  | 312 BGA-M20 VDDR1
AA9  | 313 BGA-AA9 VDDR2
G19  | 314 BGA-G19 RSV0A
H17  | 315 BGA-H17 VDD
J18  | 316 BGA-J18 VDDARR
B10  | 317 BGA-B10 VDDS15
A24  | 318 BGA-A24 VDDS18_1
R20  | 319 BGA-R20 VDDS18_2
G6   | 320 BGA-G6 VDDS18_3
K19  | 321 BGA-K19 VDDT
W12  | 322 BGA-W12 VDDT2
G20  | 323 BGA-G20 RSV0B
[Model Data]
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[End Model Data]
[End Package Model]
|   Model Cell s_ICLKRX10G_0p9
|s_iclkrx10g_0p9  [08July11 revision 1.3]
[Model]   s_iclkrx10g_0p9
Model_type   Series
Polarity   Non-Inverting
|Vinl =  1.15
|Vinh =  1.25
C_comp   0.01p   0.01p   0.01p
[Temperature Range]   25   125   -40
[Voltage Range]   0.9   0.81   0.99
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|   Model Cell s_ICLKRX10G_1
|s_iclkrx10g_1  [08July11 revision 1.3]
[Model]   s_iclkrx10g_1
Model_type   Series
C_comp   0.01p   0.01p   0.01p
[Voltage Range]   1   0.9   1.1
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| Models and submodels in the file (35): bi2c18gfz (I/O_open_drain), iclkrx10g_0p9 (Input), s_iclkrx10g_0p9 (Series), iclkrx10g_1 (Input), s_iclkrx10g_1 (Series), ihhv18g (Input), ocml10g_0p9 (Output), ocml10g_1 (Output), BC1840DGHYPBFB_WK_PD (Input), BC1840DGHYPBFB_WK_PU (Input), BC1840DGHYPBFB_DRIVER_MODE (I/O), BC1850CGHYPBFB_WK_PD (Input), BC1850CGHYPBFB_WK_PU (Input), BC1850CGHYPBFB_DRIVER_MODE (I/O), CSCDVG_SLOWEST_9MA_FT9MA (I/O), CSCDVG_SLOW_9MA_FT9MA (I/O), CSCDVG_FAST_9MA_FT9MA (I/O), CSCDVG_FASTEST_9MA_FT9MA (I/O), DIFF_FT_TH_9MA (Dynamic_clamp), CSCDDVG_SLOWEST_9MA_FT9MA_N (I/O), CSCDDVG_SLOW_9MA_FT9MA_N (I/O), CSCDDVG_FAST_9MA_FT9MA_N (I/O), CSCDDVG_FASTEST_9MA_FT9MA_N (I/O), CSCDDVG_SLOWEST_9MA_FT9MA_P (I/O), CSCDDVG_SLOW_9MA_FT9MA_P (I/O), CSCDDVG_FAST_9MA_FT9MA_P (I/O), CSCDDVG_FASTEST_9MA_FT9MA_P (I/O), CSCDVG_FASTEST_9MA (3-state), CSCDVG_FAST_9MA (3-state), CSCDVG_SLOW_9MA (3-state), CSCDVG_SLOWEST_9MA (3-state), CSCDVG_FT_TH_9MA (Dynamic_clamp), IC18GHYPBFB_WK_PD_ON (Input), IC18GHYPBFB_WK_PU_ON (Input), IC18GHYPBFB_RX_MODE (Input)
